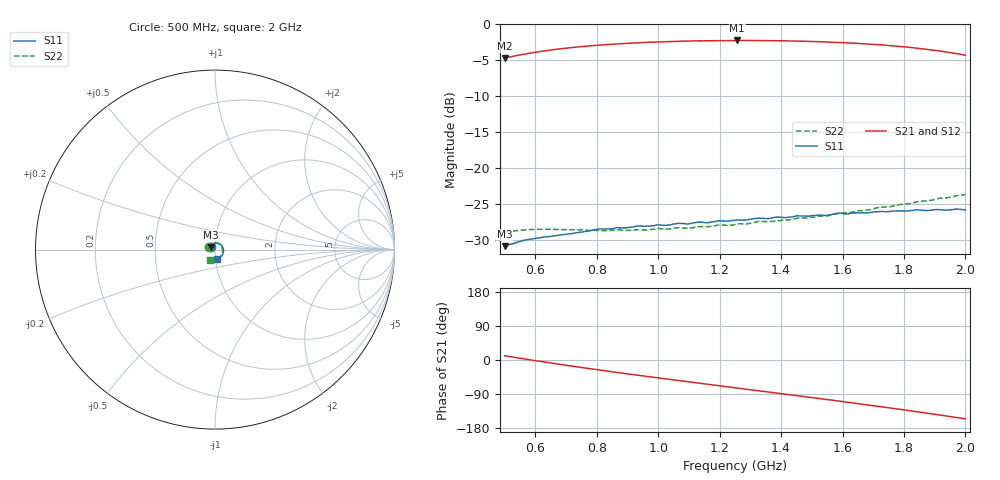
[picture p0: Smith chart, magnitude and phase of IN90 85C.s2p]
!Agilent Technologies,E8363B,SG43030131,A.07.50.48
!Agilent E8363B: A.07.50.48
!Date: Friday, October 17, 2025 03:44:07
!Correction: S11(Full 2 Port(1,2))
!S21(Full 2 Port(1,2))
!S12(Full 2 Port(1,2))
!S22(Full 2 Port(1,2))
!S2P File: Measurements: S11, S21, S12, S22:
# Hz S  dB  R 50
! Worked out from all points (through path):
!   201 points, 500 MHz to 2 GHz, reference 50 ohm
!   highest |S21| = -2.22 dB at 1.258 GHz (marker M1); lowest = -4.7 dB at 500 MHz (marker M2)
!   lowest |S11| = -30.8 dB at 500 MHz (marker M3), VSWR 1.06, Z = 47.6 + j1.41 ohm
!   |S11| at or under -10 dB: start of sweep to end of sweep
!   |S22| runs from -28.9 to -23.6 dB; largest |S21 - S12| = 0.0013
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5e8  -30.82 149.0  -4.68 11.2  -4.67 11.1  -28.85 158.4
5.675e8  -29.96 133.1  -4.09 2.4  -4.09 2.3  -28.56 142.8
6.275e8  -29.56 120.7  -3.68 -5.1  -3.68 -5.2  -28.49 130.2
6.95e8  -29.20 108.1  -3.31 -13.3  -3.31 -13.3  -28.54 116.7
7.55e8  -28.85 97.1  -3.05 -20.3  -3.07 -20.3  -28.55 103.6
8e8  -28.48 90.8  -2.90 -25.4  -2.89 -25.5  -28.65 94.4
8.75e8  -28.28 78.9  -2.67 -33.8  -2.68 -33.8  -28.55 78.7
9.575e8  -28.06 67.4  -2.49 -42.7  -2.50 -42.8  -28.60 61.9
1.0025e9  -27.87 60.9  -2.41 -47.6  -2.42 -47.5  -28.35 53.5
1.1e9  -27.72 48.4  -2.30 -57.8  -2.30 -57.8  -28.37 35.0
1.1225e9  -27.54 45.5  -2.28 -60.1  -2.28 -60.2  -28.13 31.1
1.25e9  -27.24 29.7  -2.23 -73.3  -2.22 -73.3  -27.81 8.8
1.2575e9  -27.16 28.1  -2.22 -74.1  -2.23 -74.1  -27.79 7.1
1.325e9  -26.94 20.2  -2.23 -81.0  -2.23 -81.0  -27.38 -4.3
1.3775e9  -26.83 14.7  -2.25 -86.4  -2.26 -86.4  -27.37 -12.6
1.505e9  -26.57 -0.5  -2.37 -99.6  -2.37 -99.6  -26.80 -33.5
1.625e9  -26.27 -15.5  -2.57 -112.3  -2.58 -112.3  -26.14 -53.5
1.7525e9  -26.01 -32.8  -2.93 -126.2  -2.93 -126.3  -25.36 -74.2
1.8425e9  -25.76 -47.2  -3.29 -136.5  -3.28 -136.5  -24.65 -88.5
1.88e9  -25.86 -53.2  -3.48 -140.9  -3.47 -140.8  -24.48 -94.9
1.94e9  -25.79 -64.4  -3.83 -148.0  -3.83 -148.0  -24.09 -105.3
2e9  -25.78 -77.1  -4.27 -155.4  -4.27 -155.3  -23.64 -116.1
